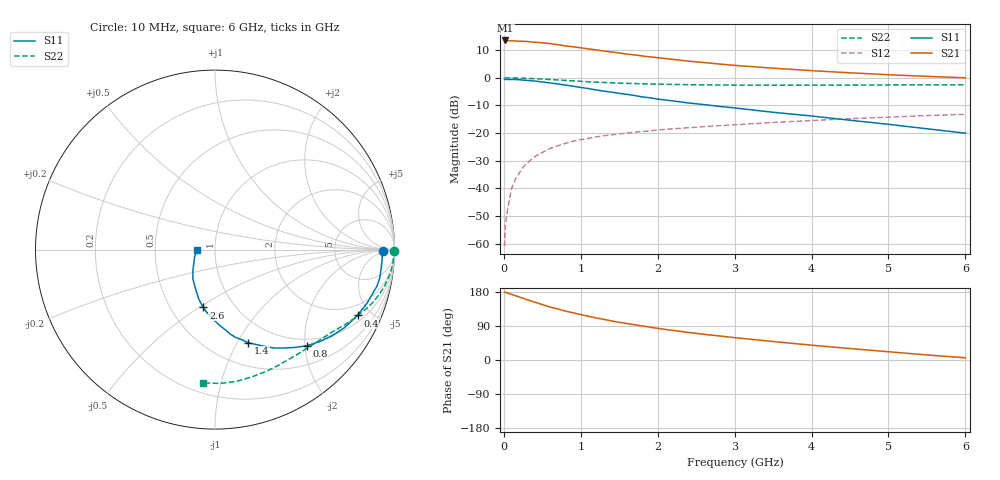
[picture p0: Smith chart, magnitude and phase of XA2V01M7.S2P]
! SIEMENS Discrete & RF Semiconductors
! BFY180
! Si NPN RF Bipolar Junction Transistor in MICRO-X
! VCE = 2 V  IC = 1.7 mA
! Common Emitter S-Parameters:  May  1997
# GHz  S  MA  R  50
!  f  S11  S21  S12  S22
! GHz  MAG  ANG  MAG  ANG  MAG  ANG  MAG  ANG
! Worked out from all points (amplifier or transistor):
!   36 points, 10 MHz to 6 GHz, reference 50 ohm
!   highest |S21| = 13.5 dB at 20 MHz (marker M1)
!   |S21| within 3 dB of that: start of sweep to 1.087 GHz
!   unconditionally stable (mu >= 1): 2.754 GHz to end of sweep
!   at 250 MHz: K = 0.12, MSG = 22.8 dB, |S12| = -32.3 dB
!   at 1.4 GHz: K = 0.67, MSG = 15.0 dB, |S12| = -20.6 dB
!   at 6 GHz: K = 1.08, MAG = 4.8 dB, |S12| = -13.2 dB
!   S11 on the Smith chart (normalised r, x): 10 MHz: 30, -5; 400 MHz: 1.32, -4.15; 800 MHz: 0.86, -2.03; 1.4 GHz: 0.75, -1.11; 2.6 GHz: 0.72, -0.52; 6 GHz: 0.82, -0.00
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0.01  0.9363 -0.6  4.681 179.3  0.0009 74.4  0.9948 -0.3
0.02  0.9313 -1.3  4.745 178.5  0.0023 91.4  0.9999 -0.7
0.05  0.9328 -3.0  4.651 176.7  0.0043 89.2  0.9954 -1.6
0.1  0.9318 -6.4  4.691 173.2  0.0099 87.4  0.9949 -3.2
0.15  0.9318 -9.7  4.645 169.8  0.0147 84.6  0.9927 -4.9
0.3  0.899 -19.2  4.545 159.2  0.0284 77.3  0.9769 -9.5
0.4  0.8749 -24.8  4.406 152.8  0.0375 74.2  0.9655 -12.4
0.5  0.8425 -31.1  4.308 146.2  0.0447 70.5  0.9488 -15.2
0.6  0.8086 -36.6  4.163 139.7  0.0526 67.1  0.9322 -17.8
0.8  0.7394 -46.4  3.785 129.1  0.0651 61.4  0.8965 -22.3
1  0.6701 -54.9  3.496 119.7  0.0764 56.6  0.865 -26.4
1.1  0.6389 -59.1  3.339 115.3  0.0804 54.5  0.85 -28.1
1.4  0.551 -70.4  2.934 103.1  0.093 49.9  0.8125 -33.1
1.5  0.5238 -73.4  2.813 99.4  0.0969 48.3  0.8024 -34.5
1.8  0.4514 -82.6  2.486 89.8  0.1072 45.2  0.78 -38.8
2  0.4124 -87.9  2.313 83.5  0.1137 43.3  0.7683 -41.5
2.2  0.382 -92.5  2.156 78.1  0.1196 41.5  0.7595 -44.3
2.6  0.3286 -101.4  1.894 67.9  0.1307 38.5  0.7465 -49.4
3.5  0.2381 -117.7  1.494 48.8  0.1556 32.5  0.7351 -60.8
4.5  0.1708 -136.2  1.233 30.2  0.182 25.2  0.7386 -74.0
5.5  0.1198 -160.8  1.063 13.3  0.2073 17.6  0.7461 -88.1
6  0.0998 -180.0  1.001 5.8  0.2186 13.3  0.7454 -95.2
